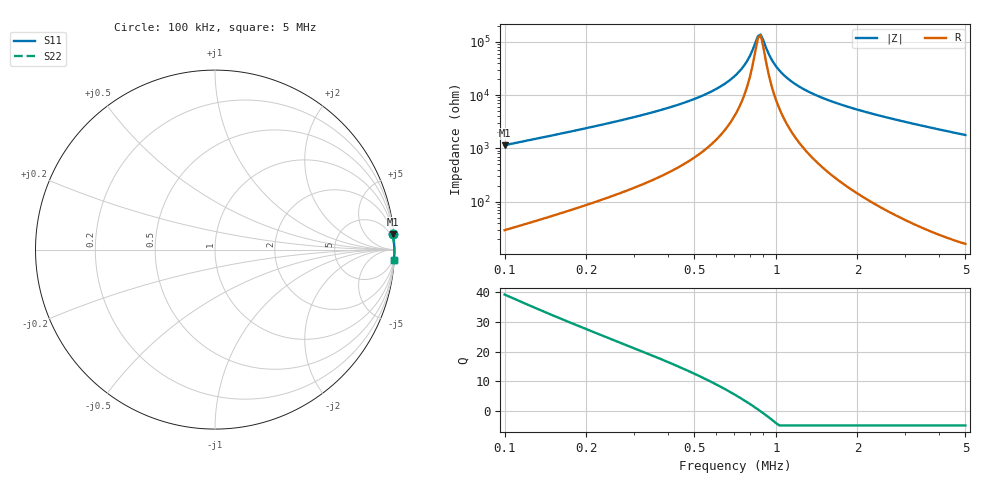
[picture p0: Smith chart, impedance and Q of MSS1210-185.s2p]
# MHz S MA R 50
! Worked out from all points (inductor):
!   172 points, 100 kHz to 5 MHz, reference 50 ohm
!   read as one part in series: L = 1.8 mH near 100 kHz
!   highest Q = 39.3 at 100 kHz (marker M1), where L = 1.82 mH
!   self-resonance near 858.9 kHz
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0.1  0.994 5.0  0.08676 -83.6  0.08676 -83.6  0.994 5.0
0.1580192  0.9968 3.1  0.05397 -85.1  0.05397 -85.1  0.9968 3.1
0.2331382  0.998 2.0  0.03517 -85.7  0.03517 -85.7  0.998 2.0
0.568981  0.9991 0.5  0.008964 -83.8  0.008964 -83.8  0.9991 0.5
0.6990645  0.9992 0.3  0.004591 -79.7  0.004591 -79.7  0.9992 0.3
0.7487274  0.9992 0.2  0.003201 -75.8  0.003201 -75.8  0.9992 0.2
0.783781  0.9992 0.1  0.002299 -70.7  0.002299 -70.7  0.9992 0.1
0.8204757  0.9993 0.1  0.001445 -59.1  0.001445 -59.1  0.9993 0.1
0.8588884  0.9993 0.0  0.0007887 -23.3  0.0007887 -23.3  0.9993 0.0
0.8787639  0.9993 -0.0  0.0007318 11.9  0.0007318 11.9  0.9993 -0.0
0.9199055  0.9993 -0.1  0.001286 56.9  0.001286 56.9  0.9993 -0.1
0.9629732  0.9993 -0.1  0.002122 71.0  0.002122 71.0  0.9993 -0.1
1.008057  0.9993 -0.2  0.003018 77.0  0.003018 77.0  0.9993 -0.2
1.079672  0.9993 -0.2  0.004404 81.3  0.004404 81.3  0.9993 -0.2
1.156374  0.9994 -0.3  0.005824 83.5  0.005824 83.5  0.9994 -0.3
1.388616  0.9994 -0.6  0.009783 86.0  0.009783 86.0  0.9994 -0.6
1.745569  0.9994 -0.9  0.01522 87.1  0.01522 87.1  0.9994 -0.9
2.096144  0.9993 -1.2  0.02014 87.4  0.02014 87.4  0.9993 -1.2
2.575376  0.9992 -1.5  0.02648 87.5  0.02648 87.5  0.9992 -1.5
3.388961  0.9989 -2.1  0.03674 87.2  0.03674 87.2  0.9989 -2.1
4.260117  0.9984 -2.7  0.04737 86.7  0.04737 86.7  0.9984 -2.7
5  0.9979 -3.2  0.05623 86.3  0.05623 86.3  0.9979 -3.2
